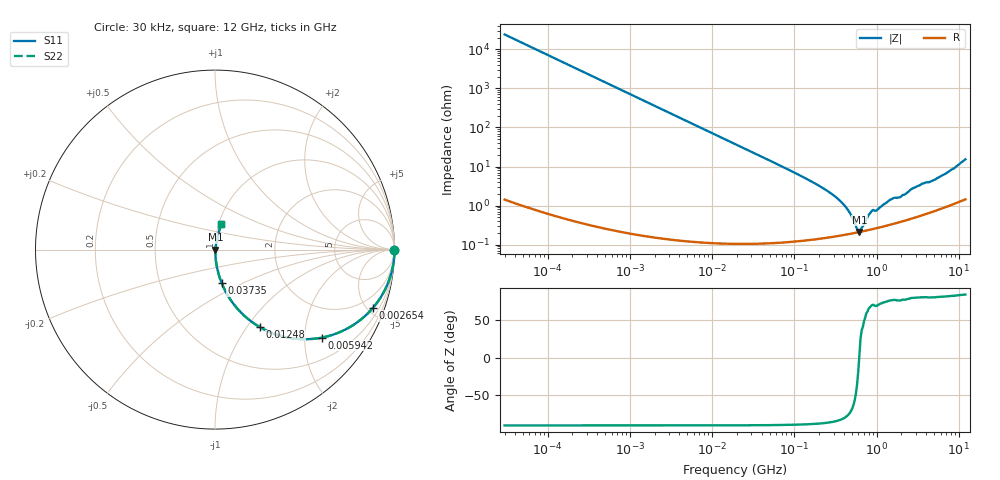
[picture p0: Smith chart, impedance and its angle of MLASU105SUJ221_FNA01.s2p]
! MLASU105SUJ221_FNA01  S-PARAMETER MODEL  ( General Type )
! Model Generated by TAIYO YUDEN Corporation (http://www.ty-top.com)
! Version 3.0
! TAIYO YUDEN Control No. 120810
! Copyright(c) 2003 TAIYO YUDEN CO.,LTD. All Rights Reserved.
! Product Description (link to TY-COMPAS)
! https://ds.yuden.co.jp/TYCOMPAS/or/detail?pn=MLASU105SUJ221JFNA01&u=M
! Products Name : Multilayer Ceramic Capacitors
! Characteristics :
!  Capacitance : 220 pF , Rated Voltage : 50V , TCC : UJ / U2J
!  Case Size : 1.0 x 0.5 / 0.039 x 0.02 [mm/inch] , Thickness : 0.5 / 0.02 [mm/inch]
!  (Conditions: Temperature = 25 degC , DC Bias Current/Voltage = 0A / 0V)
! External Node Assignments :
!  1  o---| |---o  2
! GND o---------o GND
! Frequency Range : 0.03MHz  -  12000MHz  [ 401 STEP ]
# MHz S RI R 50
! Freq[MHz].  S11 Real  S11 Imag  S21 Real  S21 Imag  S12 Real  S12 Imag  S22 Real  S22 Imag
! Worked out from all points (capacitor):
!   401 points, 30 kHz to 12 GHz, reference 50 ohm
!   read as one part in series: C = 221 pF near 32 kHz
!   lowest |Z| = 212 mohm at 617.6 MHz (marker M1)
!   series resonance near 613.9 MHz, so ESL is about 300 pH
!   S11 on the Smith chart (normalised r, x): 30 kHz: open; 2.654 MHz: 1.00, -5.42; 5.942 MHz: 1.00, -2.42; 12.48 MHz: 1.00, -1.15; 37.35 MHz: 1.00, -0.38; 12 GHz: 1.03, +0.31
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0.03  1 -0.00417  1.77e-05 0.00417  1.77e-05 0.00417  1 -0.00417
0.260295  0.9987 -0.0362  0.00131 0.0362  0.00131 0.0362  0.9987 -0.0362
0.858335  0.9859 -0.1177  0.0141 0.1177  0.0141 0.1177  0.9859 -0.1177
2.258455  0.91 -0.2859  0.09 0.2859  0.09 0.2859  0.91 -0.2859
2.65361  0.8799 -0.3248  0.1201 0.3248  0.1201 0.3248  0.8799 -0.3248
5.942454  0.5938 -0.4906  0.4062 0.4906  0.4062 0.4906  0.5938 -0.4906
12.47626  0.2494 -0.4317  0.7506 0.4317  0.7506 0.4317  0.2494 -0.4317
18.97367  0.126 -0.3304  0.874 0.3304  0.874 0.3304  0.126 -0.3304
37.34732  0.0364 -0.1846  0.9636 0.1846  0.9636 0.1846  0.0364 -0.1846
164.6252  0.00297 -0.0404  0.997 0.0404  0.997 0.0404  0.00297 -0.0404
275.7901  0.00198 -0.0208  0.998 0.0208  0.998 0.0208  0.00198 -0.0208
380.7415  0.00187 -0.0116  0.9981 0.0116  0.9981 0.0116  0.00187 -0.0116
462.0203  0.00191 -0.00676  0.9981 0.00676  0.9981 0.00676  0.00191 -0.00676
579.0248  0.00205 -0.00142  0.9979 0.00142  0.9979 0.00142  0.00205 -0.00142
617.6002  0.00211 0.000157  0.9979 -0.000157  0.9979 -0.000157  0.00211 0.000157
658.7456  0.00217 0.00163  0.9978 -0.00163  0.9978 -0.00163  0.00217 0.00163
852.6267  0.00248 0.00641  0.9975 -0.00641  0.9975 -0.00641  0.00248 0.00641
1034.641  0.00274 0.00753  0.9973 -0.00753  0.9973 -0.00753  0.00274 0.00753
1428.372  0.00336 0.0133  0.9966 -0.0133  0.9966 -0.0133  0.00336 0.0133
1909.359  0.00401 0.0157  0.996 -0.0157  0.996 -0.0157  0.00401 0.0157
5358.614  0.00982 0.048  0.9902 -0.048  0.9902 -0.048  0.00982 0.048
12000  0.0361 0.1451  0.9639 -0.1451  0.9639 -0.1451  0.0361 0.1451
